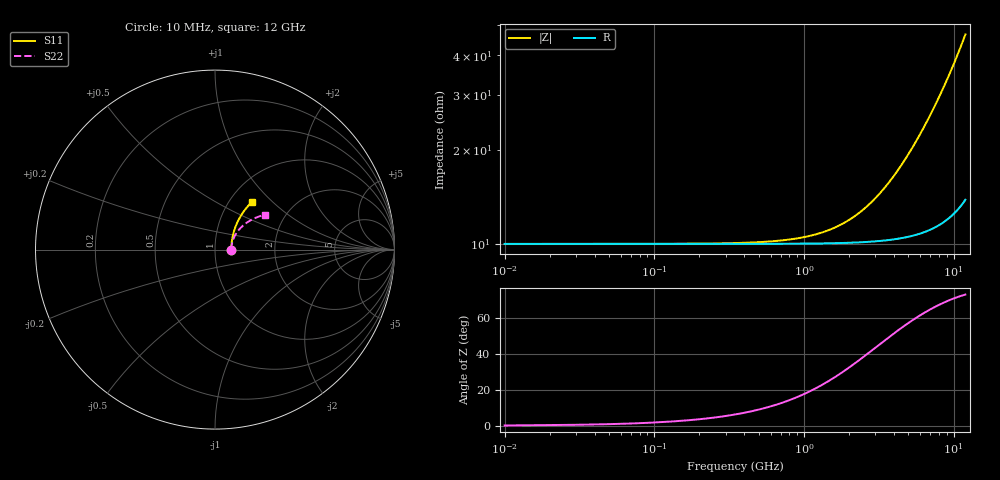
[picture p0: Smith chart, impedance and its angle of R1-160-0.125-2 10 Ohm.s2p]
!version-1
!date-03.2021
# MHz S RI R 50
!Freq ReS11 ImS11 ReS21 ImS21 ReS12 ImS12 ReS22 ImS22
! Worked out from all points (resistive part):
!   601 points, 10 MHz to 12 GHz, reference 50 ohm
!   read as one part in series: R = 10 ohm at 70 MHz
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10  0.0909 0.000213  0.9091 -0.000319  0.9091 -0.000319  0.0909 0.000193
230  0.0909 0.00491  0.909 -0.00734  0.909 -0.00734  0.091 0.00445
470  0.091 0.01  0.9089 -0.015  0.9089 -0.015  0.0912 0.00909
710  0.0912 0.0152  0.9086 -0.0226  0.9086 -0.0226  0.0915 0.0137
950  0.0915 0.0203  0.9082 -0.0303  0.9082 -0.0303  0.092 0.0184
1190  0.0918 0.0254  0.9077 -0.038  0.9077 -0.038  0.0926 0.023
1450  0.0923 0.031  0.907 -0.0462  0.907 -0.0462  0.0934 0.028
1730  0.0928 0.037  0.9061 -0.0552  0.9061 -0.0552  0.0945 0.0334
2010  0.0935 0.043  0.9051 -0.0641  0.9051 -0.0641  0.0958 0.0388
2390  0.0946 0.0511  0.9034 -0.0762  0.9034 -0.0762  0.0978 0.046
2810  0.096 0.0602  0.9012 -0.0896  0.9012 -0.0896  0.1004 0.054
3310  0.098 0.071  0.8981 -0.1055  0.8981 -0.1055  0.1041 0.0635
4010  0.1014 0.0862  0.8929 -0.1278  0.8929 -0.1278  0.1104 0.0766
5010  0.1075 0.1081  0.8836 -0.1595  0.8836 -0.1595  0.1215 0.095
6010  0.1153 0.1302  0.872 -0.1911  0.872 -0.1911  0.1353 0.1127
7010  0.1248 0.1525  0.858 -0.2224  0.858 -0.2224  0.1518 0.1298
8010  0.1362 0.175  0.8413 -0.2535  0.8413 -0.2535  0.1713 0.1459
9010  0.1498 0.1976  0.8219 -0.284  0.8219 -0.284  0.1937 0.1607
10010  0.1657 0.2203  0.7996 -0.3138  0.7996 -0.3138  0.2192 0.174
10950  0.183 0.2415  0.7757 -0.3409  0.7757 -0.3409  0.246 0.1848
11730  0.1993 0.2589  0.7536 -0.3625  0.7536 -0.3625  0.2705 0.1921
12000  0.2054 0.2649  0.7455 -0.3697  0.7455 -0.3697  0.2795 0.1943
